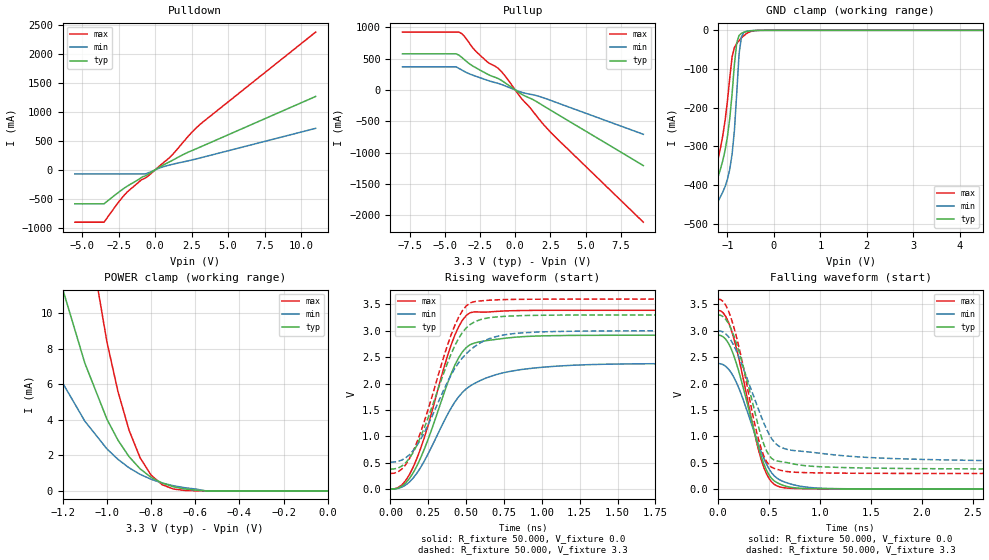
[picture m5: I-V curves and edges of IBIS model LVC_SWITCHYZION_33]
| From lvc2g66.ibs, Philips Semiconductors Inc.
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|   Model LVC_SWITCHYZION_33
[Model]   LVC_SWITCHYZION_33
Model_type   I/O
Polarity   Non-Inverting
Enable   Active-High
Vinl  =  0.8V
Vinh  =  2.0V
Vmeas =  1.5V
Cref  =  50.0pF
Rref  =  0.5k
Vref  =  0.0V
C_comp   7.68pF   5.51pF   10.52pF
[Model Spec]
| Note: The input and output voltage ratings may be exceeded if the input and
|   output current ratings are observed (please refer to the data sheet)
|   Subparameter   typ   min   max
| Thresholds
Vinh   2.0   2.0   2.0
Vinl   0.8   0.8   0.8
| Overshoot
S_overshoot_high   6.5   6.5   6.5   | Static overshoot
S_overshoot_low   -0.5   -0.5   -0.5
D_overshoot_high   7.2   7.2   7.2   | Dynamic overshoot
D_overshoot_low   -0.95   -0.9   -1.0
D_overshoot_time   3n   3n   3n
| Timing Thresholds
Vmeas   1.5   1.5   1.5
|Ambient temperature:   25   85   -40
[Temperature Range]   35   95   -30
[Voltage Range]   3.3V   3.0V   3.6V
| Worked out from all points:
|   slope of the pulldown table from 0 to 0.495 V, typ, clamps not added: 6.61 ohm
|   slope of the pullup table from 0 to 0.495 V, typ, clamps not added: 6.81 ohm
|   GND clamp passes 1 mA (typ) near -0.47 V on its own axis
|   POWER clamp passes 1 mA (typ) near -0.82 V on its own axis
|   rising waveform, R_fixture 50.000, V_fixture 0.0: 20-80 % time 225ps typ, 290ps min, 211ps max; typ from 0 V to 2.92 V
|   rising waveform, R_fixture 50.000, V_fixture 3.3: 20-80 % time 230ps typ, 269ps min, 219ps max; typ from 0.379 V to 3.3 V
|   falling waveform, R_fixture 50.000, V_fixture 0.0: 20-80 % time 243ps typ, 269ps min, 232ps max; typ from 2.92 V to 0 V
|   falling waveform, R_fixture 50.000, V_fixture 3.3: 20-80 % time 242ps typ, 305ps min, 222ps max; typ from 3.3 V to 0.379 V
|Process Range   nominal   slow   fast
[Pulldown]
| voltage   I(typ)   I(min)   I(max)
-5.5V     -585.6mA   -69.6mA    -902.4mA
-3.5V     -585.6mA   -69.6mA    -902.4mA
-2.5V     -386.3mA   -69.6mA    -556.2mA
-2.1V     -312.8mA   -69.6mA    -432.3mA
-1V       -143.2mA   -69.6mA    -184.6mA
-700mV    -106.5mA   -69.6mA    -143.4mA
-450mV    -72.08mA   -48.74mA   -100.6mA
400mV     61.46mA    40.14mA    88.42mA
1V        139.6mA    84.29mA    214.5mA
2.5V      330.5mA    169.3mA    643.6mA
3.1V      394.9mA    207mA      788.4mA
11V       1.267A     716.7mA    2.377A
[Pullup]
| voltage   I(typ)   I(min)   I(max)
-8V       574.7mA    367.6mA    920.9mA
-4.2V     574.7mA    367.6mA    920.9mA
-3.8V     519.7mA    317.8mA    897.3mA
-3.2V     408mA      250.8mA    727.9mA
-2.8V     353.6mA    217.9mA    616.5mA
-2V       254.9mA    155.3mA    450.7mA
-1.4V     198.4mA    115.1mA    374.4mA
-1V       155.1mA    88.94mA    298mA
400mV     -60.65mA   -32.89mA   -123.2mA
1.4V      -171.2mA   -84.46mA   -382mA
2.6V      -334.5mA   -174.1mA   -693.4mA
9.1V      -1.206A    -707.7mA   -2.108A
[GND_clamp]
| voltage   I(typ)   I(min)   I(max)
-5.5V     -5.637A    -5.254A    -6.275A
-1.45V    -576.2mA   -631.8mA   -539.9mA
-1.4V     -529mA     -585mA     -492.1mA
-1.3V     -438.4mA   -495.5mA   -399.9mA
-1.05V    -309.5mA   -403.4mA   -232.2mA
-950mV    -227.4mA   -358.6mA   -122.8mA
-850mV    -87.8mA    -258.8mA   -44.27mA
-800mV    -32.32mA   -162.7mA   -34.08mA
-750mV    -13.29mA   -61.33mA   -26.51mA
-700mV    -7.76mA    -17.13mA   -19.85mA
-600mV    -3.39mA    -2.491mA   -9.304mA
5.5V      1.387nA    8.75nA     187.3pA
[POWER_clamp]
| voltage   I(typ)   I(min)   I(max)
-8V       6.216A     6.248A     6.248A
-1.4V     22.23mA    14.91mA    48.63mA
-1.3V     16.38mA    9.169mA    36.1mA
-1.2V     11.34mA    6.061mA    25.02mA
-1.1V     7.186mA    3.923mA    15.68mA
-1V       4.036mA    2.364mA    8.378mA
-950mV    2.856mA    1.776mA    5.591mA
-900mV    1.932mA    1.303mA    3.421mA
-850mV    1.246mA    935.1uA    1.87mA
-750mV    444.8uA    447.7uA    352.1uA
-550mV    0A         0A         0A
0V        0A         0A         0A
[Ramp]
| variable   typ   min   max
dV/dt_r   1.750V/225.207ps   1.428V/290.078ps   2.032V/211.035ps
dV/dt_f   1.753V/241.866ps   1.493V/305.350ps   1.982V/222.251ps
R_load = 50.000
[Rising Waveform]
R_fixture   = 50.000
V_fixture   = 0.0
V_fixture_min = 0.0
V_fixture_max = 0.0
| time   V(typ)   V(min)   V(max)
0s        220.2fV    9.269pV    26.09fV
75ps      56.11mV    37.76mV    80.23mV
150ps     308.9mV    210mV      415.7mV
225ps     768mV      539.7mV    988.2mV
425ps     2.346V     1.649V     2.914V
500ps     2.68V      1.899V     3.287V
550ps     2.763V     1.995V     3.356V
850ps     2.883V     2.259V     3.382V
1.4ns     2.914V     2.365V     3.388V
8.8ns     2.917V     2.38V      3.386V
[Rising Waveform]
R_fixture   = 50.000
V_fixture   = 3.3
V_fixture_min = 3.0
V_fixture_max = 3.6
| time   V(typ)   V(min)   V(max)
0s        379mV      511.6mV    296.6mV
75ps      436.9mV    550.8mV    379.2mV
125ps     584.2mV    651mV      576mV
225ps     1.172V     1.08V      1.296V
425ps     2.717V     2.285V     3.1V
500ps     3.052V     2.563V     3.469V
575ps     3.191V     2.738V     3.559V
775ps     3.276V     2.932V     3.591V
1.2ns     3.297V     2.991V     3.599V
8.8ns     3.3V       3V         3.6V
[Falling Waveform]
R_fixture   = 50.000
V_fixture   = 0.0
V_fixture_min = 0.0
V_fixture_max = 0.0
| time   V(typ)   V(min)   V(max)
0s        2.917V     2.379V     3.386V
75ps      2.838V     2.325V     3.269V
150ps     2.549V     2.134V     2.881V
225ps     2.073V     1.806V     2.285V
375ps     942.8mV    961.1mV    907.6mV
450ps     472.9mV    576.5mV    403.3mV
525ps     201.4mV    308.8mV    136.8mV
625ps     81.28mV    156mV      33.67mV
1.2ns     6.133mV    8.803mV    4.128mV
8.8ns     4.13uV     65.03uV    45.42nV
[Falling Waveform]
R_fixture   = 50.000
V_fixture   = 3.3
V_fixture_min = 3.0
V_fixture_max = 3.6
| time   V(typ)   V(min)   V(max)
0s        3.3V       3V         3.6V
75ps      3.217V     2.942V     3.482V
150ps     2.927V     2.735V     3.097V
225ps     2.468V     2.397V     2.513V
375ps     1.343V     1.62V      1.103V
450ps     840.3mV    1.245V     620.8mV
525ps     582.6mV    957.2mV    414.5mV
650ps     512.3mV    768.4mV    341.7mV
2.4ns     384.7mV    548.3mV    297.1mV
8.8ns     379mV      511.9mV    296.6mV
